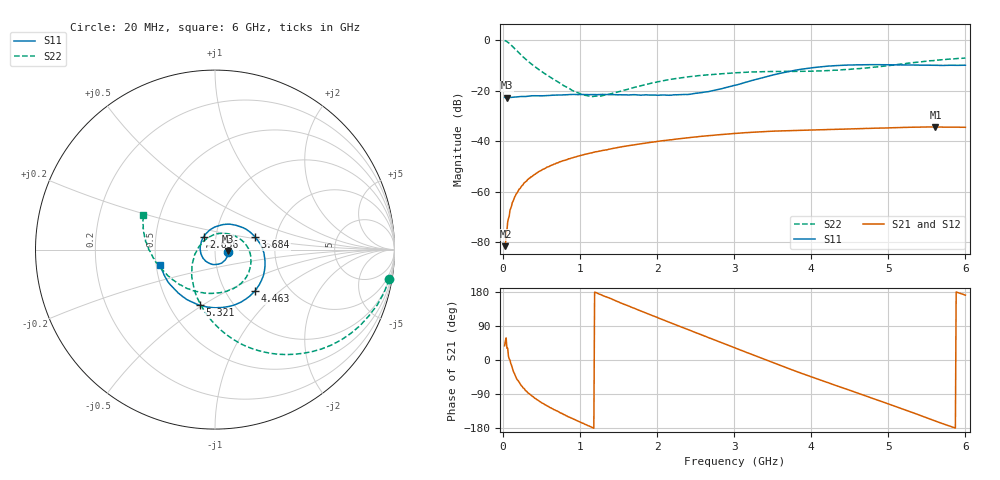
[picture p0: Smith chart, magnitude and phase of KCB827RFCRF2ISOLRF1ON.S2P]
!Agilent Technologies,E5071B,JP1KK00126,A.08.11
!Date: Tue May 06 07:31:01 2014
!Data & Calibration Information:
!Freq	S11:SOLT2(ON)	S21:SOLT2(ON)	S12:SOLT2(ON)	S22:SOLT2(ON)
# Hz S dB R 50
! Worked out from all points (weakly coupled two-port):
!   600 points, 20 MHz to 6 GHz, reference 50 ohm
!   highest |S21| = -34.40 dB at 5.611 GHz (marker M1); lowest = -81.7 dB at 29.98 MHz (marker M2)
!   lowest |S11| = -22.8 dB at 49.95 MHz (marker M3), VSWR 1.16, Z = 57.7 - j0.915 ohm
!   |S11| at or under -10 dB: start of sweep to 4.382 GHz; 5.647 GHz to 5.759 GHz (111.5 MHz wide, 1.95 % of centre); 5.918312 GHz to 5.930491 GHz (12.18 MHz wide, 0.206 % of centre)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
!   |S22| runs from -22.4 to -0.1 dB; largest |S21 - S12| = 0.00019
!   S11 on the Smith chart (normalised r, x): 20 MHz: 1.15, -0.03; 2.656 GHz: 0.87, +0.12; 3.684 GHz: 1.55, +0.23; 4.463 GHz: 1.36, -0.70; 5.321 GHz: 0.71, -0.49; 6 GHz: 0.52, -0.10
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2e7  -22.72 -11.5  -81.38 37.5  -84.44 80.9  -0.13 -9.6
2.998331e7  -22.78 -8.4  -81.66 50.4  -81.47 62.9  -0.25 -14.3
4.994992e7  -22.81 -6.3  -75.48 30.9  -74.25 34.3  -0.60 -23.3
6.991653e7  -22.79 -6.2  -70.67 9.7  -69.60 17.1  -1.02 -31.7
8.988314e7  -22.73 -6.9  -67.33 -0.7  -66.99 -0.8  -1.54 -39.4
1.49783e8  -22.57 -9.7  -62.23 -36.7  -62.26 -36.3  -3.34 -58.9
2.296494e8  -22.35 -14.1  -58.37 -65.4  -58.29 -65.5  -5.78 -78.1
3.294825e8  -22.22 -22.0  -55.06 -87.9  -54.99 -86.5  -8.51 -95.7
5.690818e8  -21.99 -38.9  -50.35 -120.6  -50.42 -120.6  -13.82 -129.2
1.018331e9  -21.55 -72.7  -45.66 -165.4  -45.63 -165.5  -21.55 159.6
1.267913e9  -21.55 -93.5  -43.88 172.7  -43.87 172.0  -22.16 107.9
2.016661e9  -21.81 -157.6  -40.09 110.6  -40.09 110.8  -16.46 23.8
2.655593e9  -20.46 132.1  -37.88 60.0  -37.89 59.8  -13.75 -12.9
3.014992e9  -17.86 88.2  -36.97 31.7  -36.97 31.5  -12.96 -32.1
3.354424e9  -14.99 49.9  -36.33 4.9  -36.32 4.5  -12.54 -49.4
3.683873e9  -12.62 17.5  -35.85 -20.8  -35.88 -21.0  -12.38 -68.0
4.013322e9  -10.94 -11.4  -35.61 -45.4  -35.64 -45.4  -12.30 -89.7
4.462571e9  -9.88 -46.2  -35.23 -77.5  -35.25 -77.6  -11.66 -121.3
5.011653e9  -9.77 -83.5  -34.77 -116.6  -34.77 -117.0  -10.04 -158.9
5.321135e9  -9.89 -105.1  -34.52 -139.3  -34.48 -139.3  -8.92 -176.4
5.610651e9  -9.98 -128.2  -34.40 -161.0  -34.38 -161.1  -8.01 169.9
6e9  -9.95 -164.2  -34.56 171.1  -34.54 171.1  -7.10 154.5
